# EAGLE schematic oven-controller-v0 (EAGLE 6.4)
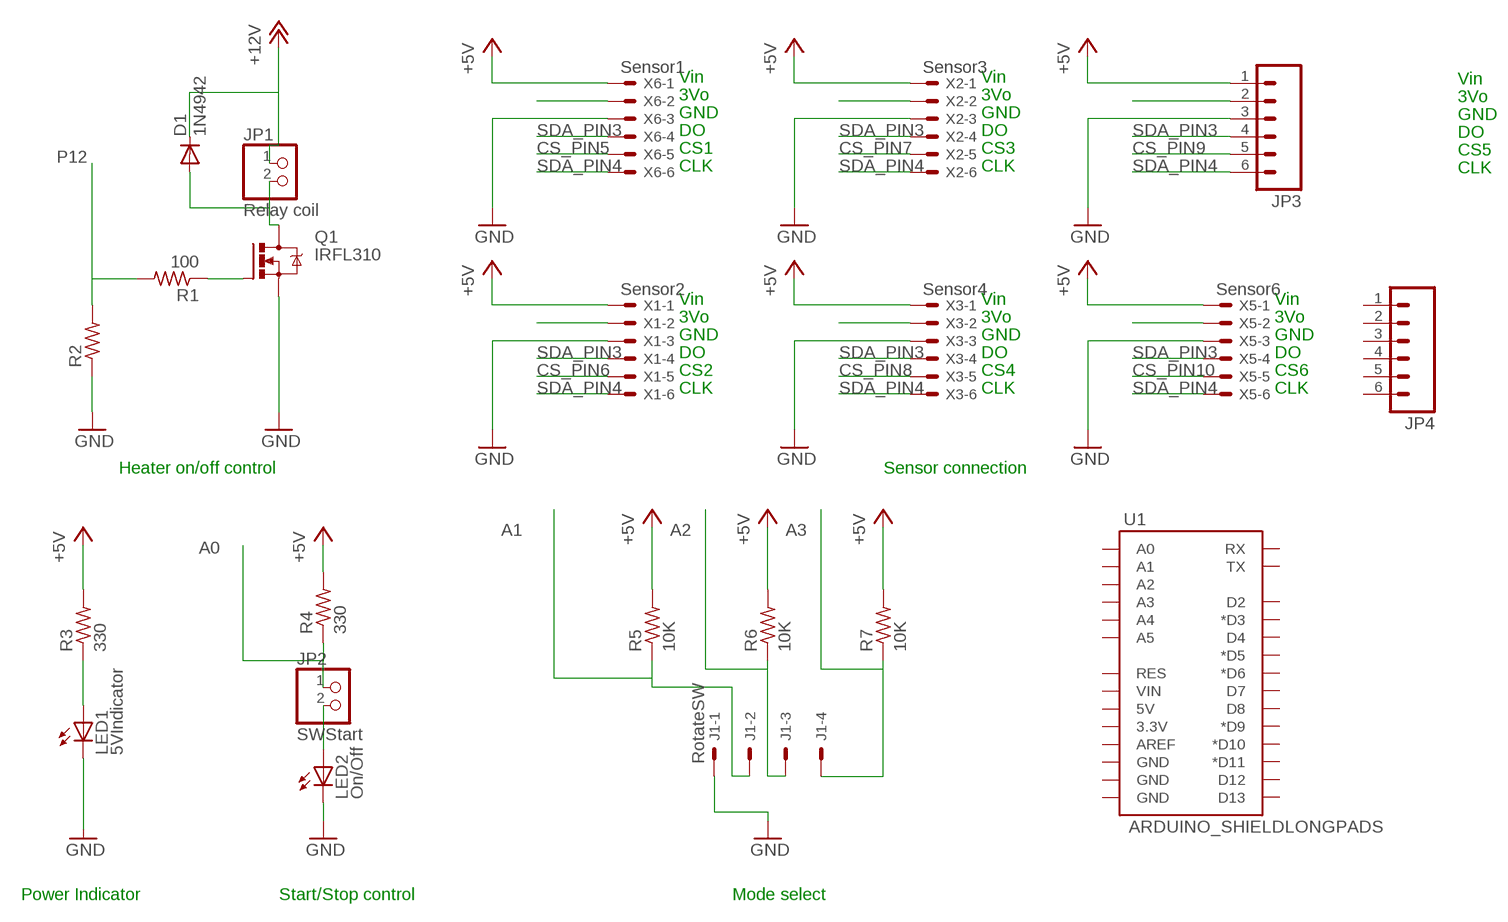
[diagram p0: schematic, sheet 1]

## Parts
D1  1N4942  [DO41-10]
J1  RotateSW  22-27-2041-04  [6410-04]
JP1  Relay coil  PINHD-1X2  [1X02]
JP2  SWStart  PINHD-1X2  [1X02]
JP3  M06LOCK_LONGPADS  [1X06_LOCK_LONGPADS]
JP4  M06LOCK_LONGPADS  [1X06_LOCK_LONGPADS]
LED1  5VIndicator  LED5MM  [LED5MM]
LED2  On/Off  LED5MM  [LED5MM]
Q1  IRFL310  IRF520  [TO220BV]
R1  100  R-US_V234/12  [V234/12]
R2  R-US_V234/12  [V234/12]
R3  330  R-US_0207/10  [0207/10]
R4  330  R-US_0207/10  [0207/10]
R5  10K  R-US_0207/10  [0207/10]
R6  10K  R-US_0207/10  [0207/10]
R7  10K  R-US_0207/10  [0207/10]
U1  ARDUINO_SHIELDLONGPADS  [DUEMILANOVE_SHIELD_LONGPADS]
X1  Sensor2  22-23-2061  [22-23-2061]
X2  Sensor3  22-23-2061  [22-23-2061]
X3  Sensor4  22-23-2061  [22-23-2061]
X5  Sensor6  22-23-2061  [22-23-2061]
X6  Sensor1  22-23-2061  [22-23-2061]

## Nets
+5V: JP3.1 R3.2 R4.2 R5.2 R6.2 R7.2 X1.1 X2.1 X3.1 X5.1 X6.1
A0: JP2.1 R4.1
A1: J1.2 R5.1
A2: J1.3 R6.1
A3: J1.4 R7.1
CS_PIN5: X6.5
CS_PIN6: X1.5
CS_PIN7: X2.5
CS_PIN8: X3.5
CS_PIN9: JP3.5
CS_PIN10: X5.5
GND: J1.1 JP3.3 LED2.K(C) Q1.S R2.1 X1.3 X2.3 X3.3 X5.3 X6.3
N$1: X1.2
N$2: Q1.G R1.1
N$3: D1.A JP1.2 Q1.D
N$4: X6.2
N$5: X2.2
N$6: X3.2
N$7: D1.C JP1.1
N$8: JP3.2
N$9: X5.2
N$10: JP2.2 LED2.A
N$11: LED1.A R3.1
N$12: LED1.K(C)
P12: R1.2 R2.2
SDA_PIN3: JP3.4 X1.4 X2.4 X3.4 X5.4 X6.4
SDA_PIN4: JP3.6 X1.6 X2.6 X3.6 X5.6 X6.6
Unconnected: JP4.1 JP4.2 JP4.3 JP4.4 JP4.5 JP4.6 U1.3.3V U1.5V U1.A0 U1.A1 U1.A2 U1.A3 U1.A4 U1.A5 U1.AREF U1.D2 U1.D3(*D3) U1.D4 U1.D5(*D5) U1.D6(*D6) U1.D7 U1.D8 U1.D9(*D9) U1.D10(*D10) U1.D11(*D11) U1.D12 U1.D13 U1.GND@0(GND) U1.GND@1(GND) U1.GND@2(GND) U1.RES U1.RX U1.TX U1.VIN

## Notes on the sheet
- Vin | Vin | Vin
- 3Vo | 3Vo | 3Vo
- GND | GND | GND
- DO | DO | DO
- CS1 | CS3 | CS5
- CLK | CLK | CLK
- Vin | Vin | Vin
- 3Vo | 3Vo | 3Vo
- GND | GND | GND
- DO | DO | DO
- CS2 | CS4 | CS6
- CLK | CLK | CLK
- Heater on/off control | Sensor connection
- Power Indicator | Start/Stop control | Mode select

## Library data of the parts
D1 = diode:1N4942: DIODE
J1 = con-molex:22-?-04: CONNECTOR wire to board 2.54 mm (.1 inch) pitch header; OC_FARNELL: unknown; OC_NEWARK: unknown
JP1 JP2 = pinhead:PINHD-1X2: PIN HEADER
JP3 JP4 = SparkFun-Connectors:M06: Header 6 Standard 6-pin 0.1" header. Use with straight break away headers (SKU : PRT-00116), right angle break away headers (PRT-00553), swiss pins (PRT-00743), machine pins (PRT-00117), and female headers (PRT-00115). Molex polarized connector foot print use with SKU : PRT-08094 with associated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
LED1 LED2 = led:LED: LED
Q1 = transistor-power:IRF520: HEXFET Power MOSFET
R1-R7 = resistor:R-US_: RESISTOR, American symbol
U1 = SparkFun-Boards:ARDUINO_SHIELD: Arduino shield footprint
X1-X3 X5 X6 = con-molex:22-23-2061: .100" (2.54mm) Center Header - 6 Pin; MF: MOLEX; MPN: 22-23-2061; OC_FARNELL: 1462922; OC_NEWARK: 27C1933

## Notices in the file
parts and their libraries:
SparkFun-Boards: Licensing: CC v3.0 Share-Alike You are welcome to use this library for commercial purposes.
